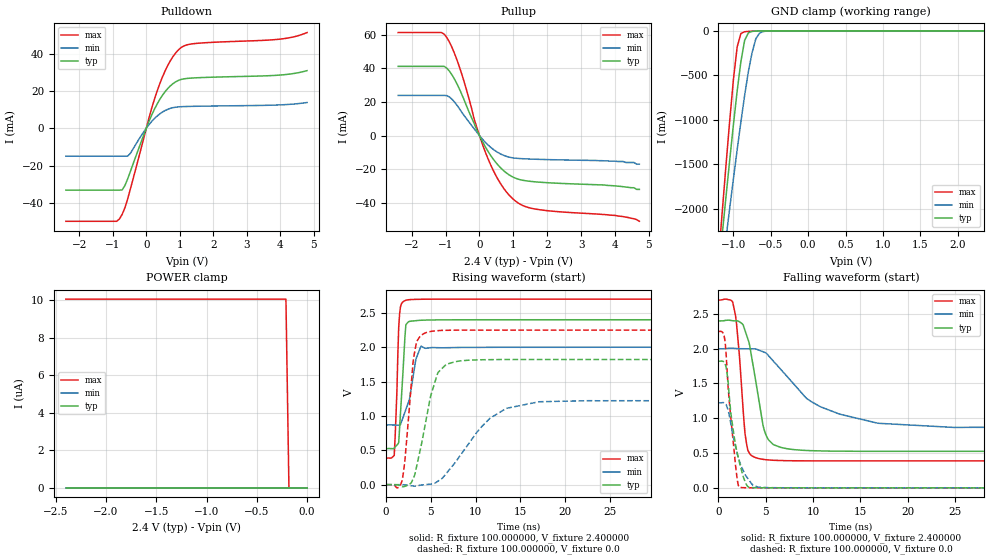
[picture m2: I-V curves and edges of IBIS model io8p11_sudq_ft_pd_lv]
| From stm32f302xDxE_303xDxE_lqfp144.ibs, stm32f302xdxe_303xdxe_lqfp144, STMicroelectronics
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|   Model io8p11_sudq_ft_pd_lv
[Model]  io8p11_sudq_ft_pd_lv
Model_type I/O
Polarity   Non-Inverting
Enable   Active-Low
Vinl =   0.720000V
Vinh =   1.680000V
Vmeas =  1.200000V
Cref =   50.000000pF
Rref =   100.000000M
Vref =   0.0V
C_comp   1.970100pF   1.887900pF   2.069400pF
[Temperature Range]   25.000000   0.125000k   -40.000000
[Pullup Reference]   2.400000V   2.000000V   2.700000V
[Pulldown Reference]   0.0V   0.0V   0.0V
[POWER Clamp Reference]   2.400000V   2.000000V   2.700000V
[GND Clamp Reference]   0.0V   0.0V   0.0V
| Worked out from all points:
|   slope of the pulldown table from 0 to 0.36 V, typ, clamps not added: 25.5 ohm
|   slope of the pullup table from 0 to 0.36 V, typ, clamps not added: 28.4 ohm
|   GND clamp passes 1 mA (typ) near -0.64 V on its own axis
|   rising waveform, R_fixture 100.000000, V_fixture 2.400000: 20-80 % time 509ps typ, 1.05ns min, 339ps max; typ from 0.525 V to 2.4 V
|   rising waveform, R_fixture 100.000000, V_fixture 0.0: 20-80 % time 1.79ns typ, 4.5ns min, 864ps max; typ from 0 V to 1.82 V
|   falling waveform, R_fixture 100.000000, V_fixture 2.400000: 20-80 % time 1.38ns typ, 6ns min, 772ps max; typ from 2.4 V to 0.525 V
|   falling waveform, R_fixture 100.000000, V_fixture 0.0: 20-80 % time 1.16ns typ, 1.4ns min, 850ps max; typ from 1.82 V to 0 V
[Pulldown]
|Voltage   I(typ)   I(min)   I(max)
-2.4V     -33.16mA   -14.98mA   -49.86mA
-880mV    -33.16mA   -14.98mA   -49.86mA
-800mV    -33.16mA   -14.98mA   -48.55mA
-640mV    -30.75mA   -14.98mA   -42.76mA
-480mV    -23.43mA   -13.57mA   -32.92mA
80mV      3.651mA    1.905mA    5.506mA
400mV     15.37mA    7.665mA    23.73mA
720mV     22.75mA    10.69mA    36.23mA
1.04V     26.18mA    11.57mA    43.27mA
1.52V     27.09mA    11.81mA    45.55mA
4V        28.55mA    12.55mA    47.81mA
4.8V      30.9mA     13.81mA    51.31mA
[Pullup]
|Voltage   I(typ)   I(min)   I(max)
-2.4V     41.23mA    23.94mA    61.35mA
-1.12V    41.23mA    23.94mA    61.35mA
-960mV    40.07mA    23.8mA     58.26mA
-800mV    35.79mA    21.42mA    51.95mA
-560mV    26.31mA    15.01mA    38.92mA
-160mV    7.338mA    4.152mA    10.02mA
240mV     -8.977mA   -5.327mA   -13.21mA
640mV     -19.51mA   -11.09mA   -29.16mA
1.04V     -25.15mA   -13.38mA   -38.61mA
1.68V     -27.56mA   -14.07mA   -43.82mA
4V        -29.9mA    -15.2mA    -47.5mA
4.72V     -32mA      -17mA      -51mA
[GND_clamp]
|Voltage   I(typ)   I(min)   I(max)
-2.4V     -9.788A    -9.782A    -9.734A
-1.2V     -2.718A    -3.021A    -2.568A
-1.15V    -2.29A     -2.675A    -2.036A
-1.1V     -1.868A    -2.333A    -1.515A
-1.05V    -1.454A    -1.995A    -1.012A
-950mV    -674.5mA   -1.337A    -180.6mA
-900mV    -345.2mA   -1.023A    -29.74mA
-850mV    -106.4mA   -726mA     -10.14mA
-750mV    -6.411mA   -244mA     -4.042mA
-700mV    -2.572mA   -88.62mA   -2.346mA
-600mV    -429.6uA   -7.75mA    -383.5uA
2.35V     59.77uA    46.33uA    66.89uA
[POWER_clamp]
|Voltage   I(typ)   I(min)   I(max)
-2.4V     0A         0A         10.06uA
-210mV    0A         0A         10.06uA
-180mV    0A         0A         0A
0V        0A         0A         0A
[Ramp]
| variable   typ   min   max
dV/dt_r  1.09218/1.79238n   0.73266/4.49807n   1.34886/0.85997n
dV/dt_f  1.12444/1.38128n   0.67760/5.98085n   1.38699/0.77171n
R_load = 100.000000
[Rising Waveform]
R_fixture= 100.000000
V_fixture= 2.400000
V_fixture_min= 2.000000
V_fixture_max= 2.700000
|time   V(typ)   V(min)   V(max)
0s        524.8mV    868.7mV    387.2mV
900.9ps   532.4mV    867.1mV    423.6mV
1.201ns   575.3mV    865.9mV    1.359V
1.401ns   611.4mV    865.5mV    2.286V
1.602ns   1.042V     875.4mV    2.59V
2.202ns   2.327V     1.094V     2.683V
2.603ns   2.374V     1.24V      2.691V
3.303ns   2.385V     1.812V     2.695V
3.904ns   2.392V     2.015V     2.697V
49.85ns   2.399V     1.999V     2.699V
[Rising Waveform]
R_fixture= 100.000000
V_fixture= 0.0
V_fixture_min= 0.0
V_fixture_max= 0.0
|time   V(typ)   V(min)   V(max)
0s        -34.41uV   -16.09uV   -30.77uV
1.802ns   -29.45mV   -740.5uV   67.35mV
3.103ns   111mV      -21.8mV    1.872V
3.403ns   265.9mV    -17.88mV   2.083V
4.505ns   973.4mV    1.615mV    2.214V
5.706ns   1.601V     43.39mV    2.239V
6.707ns   1.75V      161.3mV    2.245V
10.71ns   1.817V     848.5mV    2.248V
13.51ns   1.82V      1.112V     2.248V
49.85ns   1.82V      1.221V     2.248V
[Falling Waveform]
R_fixture= 100.000000
V_fixture= 2.400000
V_fixture_min= 2.000000
V_fixture_max= 2.700000
|time   V(typ)   V(min)   V(max)
0s        2.399V     1.999V     2.699V
1.502ns   2.401V     2.006V     2.669V
1.902ns   2.399V     2.002V     2.364V
2.903ns   2.22V      1.998V     687.3mV
4.004ns   1.477V     1.993V     430.5mV
5.205ns   707.5mV    1.911V     401.7mV
7.508ns   556.9mV    1.561V     389.5mV
10.81ns   530.5mV    1.163V     387.2mV
16.82ns   524.9mV    928.9mV    387.2mV
49.85ns   524.8mV    868.7mV    387.2mV
[Falling Waveform]
R_fixture= 100.000000
V_fixture= 0.0
V_fixture_min= 0.0
V_fixture_max= 0.0
|time   V(typ)   V(min)   V(max)
0s        1.82V      1.221V     2.248V
700.7ps   1.782V     1.213V     2.099V
1.101ns   1.38V      1.068V     1.302V
1.301ns   1.08V      922.8mV    1.007V
1.802ns   621.8mV    592.1mV    322mV
2.102ns   428.2mV    431.4mV    33.52mV
2.302ns   319.1mV    346.1mV    4.266mV
3.103ns   16.96mV    133.5mV    1.213mV
4.605ns   776.8uV    5.445mV    417.8uV
49.85ns   -34.41uV   -16.09uV   -30.77uV
